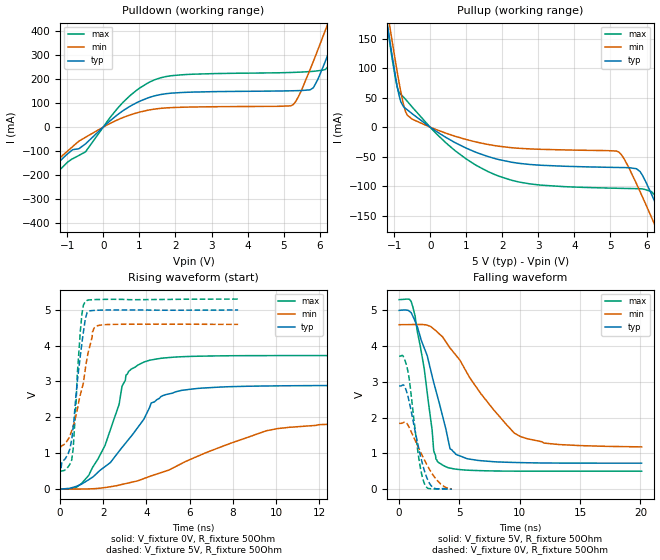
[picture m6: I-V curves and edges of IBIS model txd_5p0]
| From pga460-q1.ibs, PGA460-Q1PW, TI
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|   txd_5p0 Model
[Model]   txd_5p0
Model_type   Output
Polarity   Non-Inverting
Vmeas = 2.5
Vref = 0
Cref = 2pF
Rref = 600
|   typ   min   max
|   (nom PVT)   (fast PVT)   (slow PVT)
C_comp   1.508e-12   1.508e-12   1.546e-12
| Where nom  PVT is Nominal Process, 5V, 27C
|   Fast PVT is Strong Process,  5.3V, -40C
|   Slow PVT is Weak Process,   4.6V, 125C
[Voltage Range]   5   4.6   5.3
|Junction Temperature
[Temperature Range]   27   125   -40
[Pullup Reference]   5   4.6   5.3
[Pulldown Reference]   0   0   0
[Power Clamp Reference]   5   4.6   5.3
[GND Clamp Reference]   0   0   0
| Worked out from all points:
|   slope of the pulldown table from 0 to 0.75 V, typ, clamps not added: 8.62 ohm
|   slope of the pullup table from 0 to 0.75 V, typ, clamps not added: 26.8 ohm
|   falling waveform, V_fixture 5V, R_fixture 50Ohm: 20-80 % time 2.08ns typ, 4.45ns min, 1.23ns max; typ from 5 V to 0.729 V
|   rising waveform, V_fixture 0V, R_fixture 50Ohm: 20-80 % time 2.19ns typ, 4.61ns min, 1.31ns max; typ from 0 V to 2.89 V
|   rising waveform, V_fixture 5V, R_fixture 50Ohm: 20-80 % time 446ps typ, 688ps min, 289ps max; typ from 0.729 V to 4.99 V
|   falling waveform, V_fixture 0V, R_fixture 50Ohm: 20-80 % time 1.12ns typ, 1.68ns min, 812ps max; typ from 2.89 V to 0.002 V
[Pulldown]
|   Voltage   I(typ)   I(min)   I(max)
-5V       -690.3mA   -655.7mA   -737.5mA
-1.734V   -216.8mA   -197.3mA   -256.9mA
-496.6mV  -69.65mA   -42.1mA    -102.8mA
3.2mV     1.204mA    670.3uA    1.886mA
702.8mV   83.56mA    48.77mA    126.1mA
1.461V    131.6mA    75.95mA    199.1mA
5.197V    151.1mA    88.58mA    227.3mA
5.405V    151.9mA    125mA      228.4mA
5.825V    164mA      273.6mA    232.1mA
6.231V    302.5mA    431.8mA    252mA
6.766V    519.3mA    646.8mA    458.9mA
10V       1.873A     1.995A     1.861A
[Pullup]
|   Voltage   I(typ)   I(min)   I(max)
-5V       1.779A     1.744A     1.832A
-1.295V   216.4mA    238.1mA    214.8mA
-1.095V   135.3mA    159.6mA    130.4mA
-915mV    68.72mA    92.7mA     67.06mA
-639.2mV  29.39mA    20.23mA    43.87mA
662.6mV   -25.4mA    -14.92mA   -38.61mA
1.905V    -55.01mA   -32.37mA   -83.15mA
5.24V     -68.39mA   -42.63mA   -103.6mA
5.82V     -75.25mA   -109.2mA   -104.4mA
6.353V    -143.9mA   -183.1mA   -131.3mA
6.734V    -199.6mA   -237.3mA   -187.6mA
10V       -697.5mA   -711.1mA   -715.7mA
[Ramp]
R_load = 50
|   typ   min   max
dV/dt_r   1.73266/2.34534e-09   1.10554/4.19224e-09   2.23344/1.38791e-09
dV/dt_f   2.56276/1.93654e-09   2.05437/4.04983e-09   2.87738/1.1547e-09
[Falling Waveform]
V_fixture = 5V
V_fixture_min = 4.6V
V_fixture_max = 5.3V
R_fixture = 50Ohm
|   Time   V(typ)   V(min)   V(max)
0s        5V         4.6V       5.3V
861.6ps   4.973V     4.603V     5.308V
1.325ns   4.692V     4.605V     4.836V
2.082ns   3.947V     4.6V       3.363V
2.867ns   2.982V     4.48V      1.067V
3.297ns   2.444V     4.352V     739.4mV
4.217ns   1.13V      3.95V      590.7mV
4.669ns   986.4mV    3.761V     563.1mV
10.06ns   744.6mV    1.471V     505.2mV
20.1ns    728.6mV    1.184V     504.2mV
[Rising Waveform]
V_fixture = 0V
V_fixture_min = 0V
V_fixture_max = 0V
R_fixture = 50Ohm
|   Time   V(typ)   V(min)   V(max)
0s        282.7pV    1.119nV    331.3pV
1.325ns   259.3mV    1.675mV    380.7mV
2.082ns   626.3mV    40.24mV    1.219V
2.732ns   1.054V     108mV      2.361V
3.049ns   1.292V     152.2mV    3.177V
3.902ns   1.976V     295.4mV    3.546V
4.217ns   2.399V     365.7mV    3.601V
5.618ns   2.751V     706.6mV    3.69V
10.06ns   2.877V     1.684V     3.722V
18.7ns    2.888V     1.84V      3.722V
[Rising Waveform]
V_fixture = 5V
V_fixture_min = 4.6V
V_fixture_max = 5.3V
R_fixture = 50Ohm
|   Time   V(typ)   V(min)   V(max)
0s        728.6mV    1.176V     504.2mV
34.27ps   545.7mV    1.177V     502.5mV
533.1ps   1.371V     1.625V     803.2mV
605.4ps   1.733V     1.756V     1.129V
936.4ps   3.725V     2.633V     4.416V
1.076ns   4.375V     2.96V      5.127V
1.191ns   4.799V     3.454V     5.238V
1.5ns     4.979V     4.391V     5.282V
1.727ns   4.987V     4.557V     5.287V
8.248ns   4.994V     4.592V     5.299V
[Falling Waveform]
V_fixture = 0V
V_fixture_min = 0V
V_fixture_max = 0V
R_fixture = 50Ohm
|   Time   V(typ)   V(min)   V(max)
0s        2.888V     1.843V     3.722V
322.1ps   2.915V     1.858V     3.724V
710.4ps   2.621V     1.803V     3.322V
933.1ps   2.288V     1.654V     2.822V
1.591ns   1.193V     1.17V      955.8mV
1.839ns   830.6mV    993.1mV    466.7mV
2.111ns   498.2mV    807.4mV    143.1mV
2.778ns   54.3mV     411.6mV    9.608mV
3.43ns    7.241mV    148.8mV    14.32mV
4.369ns   2.076mV    8.706mV    6.574mV
